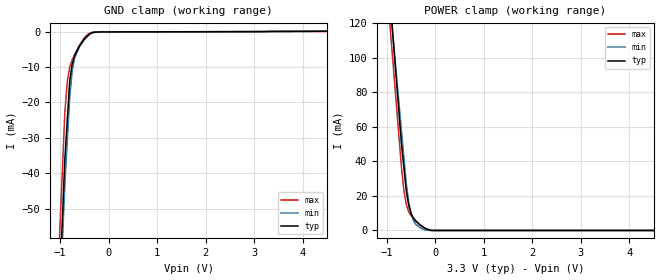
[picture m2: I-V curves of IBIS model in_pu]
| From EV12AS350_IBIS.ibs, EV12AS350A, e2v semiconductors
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[Model] in_pu
Model_type Input
Vinl = 1.15500V
Vinh = 2.14500V
C_comp 487.000fF 444.000fF 530.000fF
| variable typ   min   max
[Voltage Range] 3.30000V 3.20000V 3.40000V
[POWER Clamp Reference] 3.30000V 3.20000V 3.40000V
[GND Clamp Reference] 0.00000V 0.00000V 0.00000V
[Temperature Range]   25   110   -40
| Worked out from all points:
|   GND clamp passes 1 mA (typ) near -0.42 V on its own axis
|   POWER clamp passes 1 mA (typ) near -0.19 V on its own axis
[GND Clamp]
-3.3V     -841.6mA   -815.5mA   -791.2mA
-900mV    -36.1mA    -43.23mA   -22.88mA
-850mV    -25.11mA   -30.96mA   -14.18mA
-800mV    -14.11mA   -18.68mA   -10.08mA
-750mV    -9.24mA    -11.39mA   -7.934mA
-700mV    -6.825mA   -7.585mA   -6.569mA
-600mV    -4.145mA   -4.319mA   -3.84mA
-500mV    -2.121mA   -2.285mA   -1.778mA
-450mV    -1.441mA   -1.59mA    -1.033mA
-350mV    -375.5uA   -468.1uA   -224.5uA
-150mV    -82.94uA   -62.8uA    -68.61uA
6.6V      200.2uA    307.2uA    103.9uA
[POWER Clamp]
-3.3V     978.3mA    862.7mA    940.5mA
-800mV    85.99mA    88.99mA    71.49mA
-700mV    50.3mA     58.04mA    36.73mA
-650mV    36.66mA    42.57mA    23.49mA
-600mV    23.02mA    27.09mA    15.08mA
-550mV    14.58mA    16.62mA    10.78mA
-500mV    9.635mA    10.01mA    8.454mA
-450mV    7.035mA    5.653mA    6.871mA
-300mV    2.907mA    1.301mA    2.746mA
-200mV    1.107mA    238.6uA    830.1uA
-50mV     0A         0A         40.27uA
6.6V      0A         0A         0A
